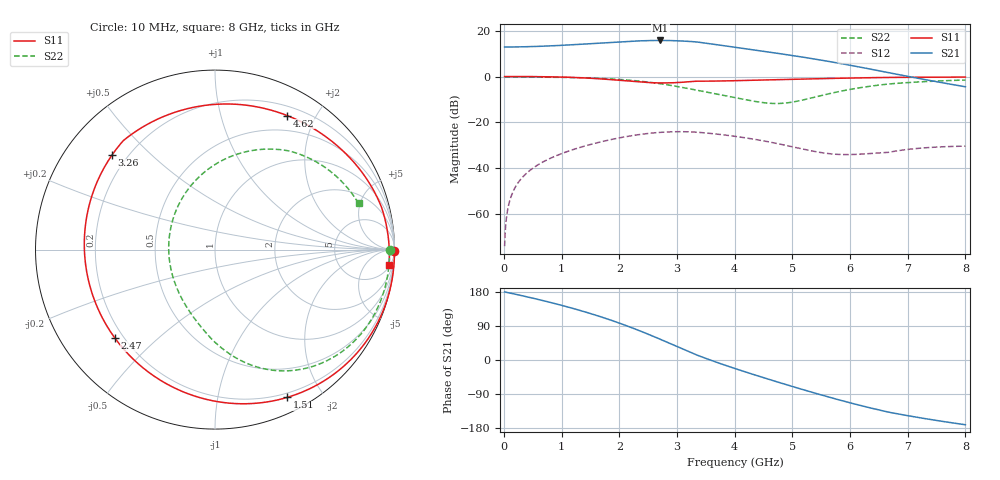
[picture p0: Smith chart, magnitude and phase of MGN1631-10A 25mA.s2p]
! Port[1] = GATE
! Port[2] = DRAIN
! [Type]  S-parameter s2p file touchstone ver. 1.0
! [Object]  MGN1631-10A
! [Bias]  25 mA
! [Version]  1.0
! [Date]  Thu May 19 10:15:03 2026
! [Source]  This file was created in JSC "ICC Milandr".
! [Disclaimer] Property of JSC "ICC Milandr". Unauthorized reproduction and/or distribution is strictly prohibited.
!  The file and the data are provided "AS IS" and with all faults and disclaim all warranties, express and implied, including
!  without limitation any implied warranties of merchantability, fitness for a particular purpose.
!  JSC "ICC Milandr" assumes no liability for:
!  1) the accuracy of the data provided;
!  2) the proper functioning of this data;
!  3) infringement of patents, copyrights or intellectual property rights resulting from the use of this data.
!  JSC "ICC Milandr" reserves the right to make changes to the products and the data without prior notice.
!  Please, be aware that your receipt and use of the file provided shall serve as acceptance of these terms and conditions.
!  If you do not accept these terms, you should return or destroy this file and any other accompanying information immediately.
# Hz S MA R 12.5
! freq  S11mag  S11ang  S21mag  S21ang  S12mag  S12ang  S22mag  S22ang
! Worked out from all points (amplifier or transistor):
!   800 points, 10 MHz to 8 GHz, reference 12.5 ohm
!   highest |S21| = 15.8 dB at 2.71 GHz (marker M1)
!   |S21| within 3 dB of that: start of sweep to 4.013 GHz
!   unconditionally stable (mu >= 1): 4.736 GHz to 6.49 GHz
!   at 1.34 GHz: K = 0.27, MSG = 22.5 dB, |S12| = -30.8 dB
!   at 4.01 GHz: K = 0.73, MSG = 19.5 dB, |S12| = -26.1 dB
!   at 8 GHz: K = 0.52, MSG = 13.0 dB, |S12| = -30.4 dB
!   S11 on the Smith chart (normalised r, x): 10 MHz: open; 1.51 GHz: 0.15, -1.59; 2.47 GHz: 0.17, -0.37; 3.26 GHz: 0.14, +0.38; 4.62 GHz: 0.31, +1.63; 8 GHz: 6, -21
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1e7  1 -0.3  4.42 179.6  0.0001976 85.8  0.9725 -0.2
1.1e8  1.001 -3.9  4.422 176.4  0.002159 86.6  0.9729 -2.2
3.1e8  1 -11.1  4.459 169.8  0.006124 81.1  0.9729 -6.2
8.8e8  0.9829 -33.3  4.726 149.0  0.01811 63.3  0.9646 -18.3
1.35e9  0.9391 -55.2  5.094 129.4  0.02915 46.2  0.9415 -29.3
1.51e9  0.9167 -63.9  5.243 122.1  0.03316 39.8  0.9286 -33.4
1.78e9  0.8708 -80.5  5.51 108.9  0.04013 28.1  0.899 -40.7
2.06e9  0.8159 -101.0  5.783 94.0  0.04734 14.7  0.8557 -48.9
2.27e9  0.7755 -119.1  5.961 82.0  0.05243 3.8  0.8133 -55.5
2.47e9  0.7443 -138.6  6.086 69.9  0.05667 -7.2  0.7648 -62.0
2.68e9  0.7267 -160.9  6.143 56.6  0.06011 -19.5  0.706 -69.0
2.71e9  0.7259 -164.2  6.144 54.6  0.06049 -21.3  0.6971 -70.0
3e9  0.7396 163.9  6.047 35.6  0.06254 -38.9  0.6074 -79.8
3.26e9  0.7789 137.5  5.803 18.5  0.0617 -54.9  0.5278 -88.7
3.63e9  0.7959 108.8  5.086 -3.0  0.05647 -72.1  0.4304 -101.4
4.01e9  0.8123 86.9  4.355 -22.8  0.0494 -84.9  0.3468 -119.0
4.31e9  0.8295 73.3  3.852 -37.5  0.04332 -92.3  0.2929 -139.1
4.62e9  0.8482 61.7  3.389 -52.3  0.03686 -97.3  0.2603 -167.5
5.34e9  0.8916 41.2  2.466 -85.2  0.02371 -93.8  0.3434 121.4
5.96e9  0.9259 27.5  1.805 -111.4  0.01976 -73.1  0.5133 82.7
6.67e9  0.9573 14.3  1.215 -137.7  0.02217 -58.4  0.6882 52.9
8e9  0.974 -5.0  0.5982 -170.9  0.03025 -79.4  0.8406 17.8
